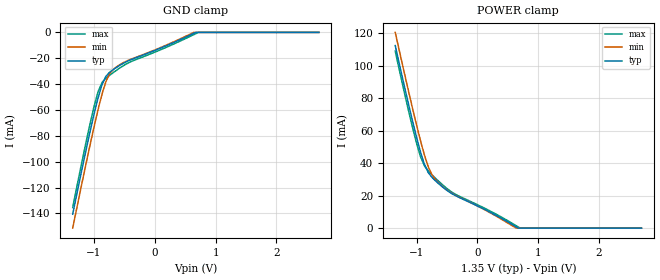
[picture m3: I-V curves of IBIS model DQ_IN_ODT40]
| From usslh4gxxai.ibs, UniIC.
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| MODEL DQ_IN_ODT40 (Data Input with 40ohm ODT, 800-2133Mbps)
[Model]   DQ_IN_ODT40
Model_type   Input
Vinl = 545.000mV
Vinh = 805.000mV
|   typ   min   max
|C_comp   0.965pF   0.916pF   1.023pF
C_comp_power_clamp   0.4825pF   0.4580pF   0.5115pF
C_comp_gnd_clamp   0.4825pF   0.4580pF   0.5115pF
| Note: C_comp changes when the ODT circuit is enabled.
[Model Spec]
| Input threshold voltage corners
Vinl   0.5450V   0.5115V   0.5825V
Vinh   0.8050V   0.7715V   0.8425V
| Dynamic Overshoot Parameters from DDR3L Specification
|D_overshoot_ampl_h   0.40   NA   NA
|D_overshoot_ampl_l   0.40   NA   NA
|D_overshoot_area_h   0.11n   NA   NA
|D_overshoot_area_l   0.11n   NA   NA
[Receiver Thresholds]
Vth   =  0.675V
Vth_min  =  0.6615V
Vth_max  =  0.6885V
Vinh_ac  =  0.130V
Vinh_dc  =  0.090V
Vinl_ac  = -0.130V
Vinl_dc  = -0.090V
Tslew_ac =  5.000ns |Not specified, so set to high value
Threshold_sensitivity = 0.50
Reference_supply Power_clamp_ref
[Voltage Range]   1.3500V   1.2830V   1.4250V
[POWER Clamp Reference]   1.3500V   1.2830V   1.4250V
[Temperature Range]   45.0   95.0   -40.0
[GND Clamp]
|   Voltage   I(typ)   I(min)   I(max)
-1.35V    -140.6mA   -151.4mA   -135.4mA
-1.075V   -78.79mA   -89.12mA   -72.64mA
-1.005V   -64.28mA   -74.23mA   -58.32mA
-935mV    -51mA      -60.09mA   -46.14mA
-875mV    -41.28mA   -49.01mA   -39.62mA
-800mV    -33.79mA   -37.59mA   -35.32mA
-745mV    -30.93mA   -32.17mA   -33.27mA
-640mV    -27.38mA   -26.98mA   -29.63mA
-400mV    -21.26mA   -20.92mA   -22.77mA
640mV     -769.1uA   -43.13uA   -1.774mA
720mV     0A         0A         0A
2.7V      0A         0A         0A
[POWER Clamp]
|   Voltage   I(typ)   I(min)   I(max)
-1.35V    112.5mA    120.7mA    109.1mA
-1.075V   67.44mA    75.31mA    63.48mA
-935mV    47.05mA    54.01mA    44.1mA
-875mV    39.82mA    45.82mA    38.92mA
-810mV    34.41mA    38.26mA    35.42mA
-750mV    31.45mA    33.22mA    33.03mA
-690mV    29.22mA    29.94mA    30.83mA
-550mV    24.74mA    24.87mA    26.01mA
-340mV    19.7mA     19.9mA     20.47mA
640mV     765.8uA    22.39uA    1.479mA
705mV     0A         0A         0A
2.7V      0A         0A         0A
